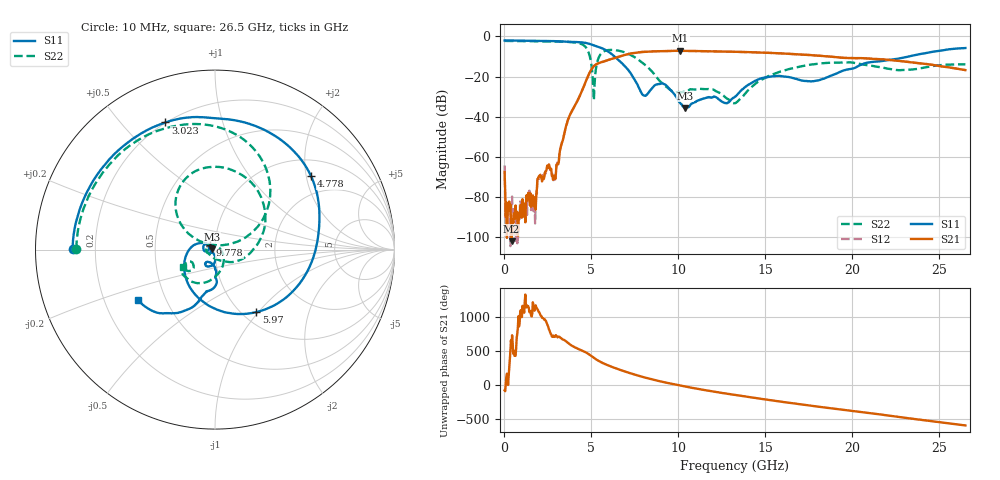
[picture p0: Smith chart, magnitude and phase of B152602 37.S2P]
!  2-Port S-parameters saved by WinCal
! VAR MeasName=S-Parameters (CALIBRATED_DATA) read from VNA (N5242A)
! VAR MeasDate=2016-1-5 16:31:34
! VAR NAME=B152602 37
! VAR FILENAME=B152602 37.S2P
! VAR DATE=2016-1-5 16:31:34
! VAR PHYS_PORTS=1,2
# Hz S DB R 50
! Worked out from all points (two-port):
!   801 points, 10 MHz to 26.5 GHz, reference 50 ohm
!   highest |S21| = -7.16 dB at 10.11 GHz (marker M1); lowest = -101.9 dB at 407.4 MHz (marker M2)
!   |S21| within 3 dB of the highest: 6.539 GHz to 18.88 GHz (12.34 GHz wide, 97.1 % of centre)
!   lowest |S11| = -35.6 dB at 10.37 GHz (marker M3), VSWR 1.03, Z = 48.4 + j0.259 ohm
!   |S11| at or under -10 dB: 6.336 GHz to 23.24 GHz (16.91 GHz wide, 114 % of centre)
!   |S22| runs from -33.3 to -2.2 dB; largest |S21 - S12| = 0.0022
!   S11 on the Smith chart (normalised r, x): 10 MHz: 0.12, +0.00; 3.023 GHz: 0.20, +0.66; 4.778 GHz: 1.42, +2.13; 5.97 GHz: 1.16, -0.98; 9.778 GHz: 0.95, +0.05; 26.5 GHz: 0.35, -0.26
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1e7  -2.01 179.7  -67.51 -82.6  -64.19 -173.0  -2.24 179.8
4.0735e8  -2.04 171.6  -101.92 -169.2  -83.03 -177.1  -2.25 173.7
1.698738e9  -2.20 144.7  -84.71 22.9  -87.06 81.2  -2.36 153.3
2.029862e9  -2.23 137.2  -69.22 -28.6  -69.31 -26.9  -2.40 147.7
3.023238e9  -2.38 111.3  -63.59 -11.7  -64.13 -8.0  -2.53 128.2
3.652375e9  -2.69 91.0  -41.50 -103.9  -41.55 -104.5  -2.74 111.9
4.447075e9  -2.97 57.1  -27.27 145.6  -27.28 145.7  -3.86 77.0
4.7782e9  -3.43 37.6  -20.29 101.4  -20.31 101.5  -6.76 47.8
5.142438e9  -4.45 14.0  -14.78 35.8  -14.79 36.0  -31.75 102.6
5.473562e9  -5.42 -10.2  -13.14 -17.5  -13.13 -17.4  -9.60 131.8
5.97025e9  -7.58 -56.5  -11.70 -76.1  -11.69 -76.1  -6.79 98.5
7.062962e9  -16.14 -173.2  -8.89 -176.4  -8.89 -176.4  -8.45 45.5
7.990112e9  -29.25 164.9  -7.72 111.8  -7.71 111.9  -13.50 -0.2
8.851038e9  -23.69 174.3  -7.34 56.2  -7.33 56.2  -21.43 -50.8
9.778188e9  -28.85 138.0  -7.18 4.5  -7.19 4.6  -27.73 -116.3
1.010931e10  -33.18 147.0  -7.16 -12.8  -7.16 -12.8  -27.75 -138.8
1.037421e10  -35.55 170.8  -7.19 -26.2  -7.20 -26.2  -27.54 -148.8
1.3255e10  -30.02 -95.0  -7.65 -150.5  -7.65 -150.4  -33.26 48.3
1.494374e10  -20.50 -103.8  -8.12 145.3  -8.10 145.2  -20.78 -60.1
1.769208e10  -22.29 -109.5  -9.36 48.6  -9.35 48.8  -13.96 -111.7
2.209604e10  -11.74 -104.0  -11.68 -94.5  -11.62 -94.6  -16.15 -155.3
2.65e10  -5.78 -146.9  -16.76 120.9  -16.76 120.4  -13.92 -150.8
